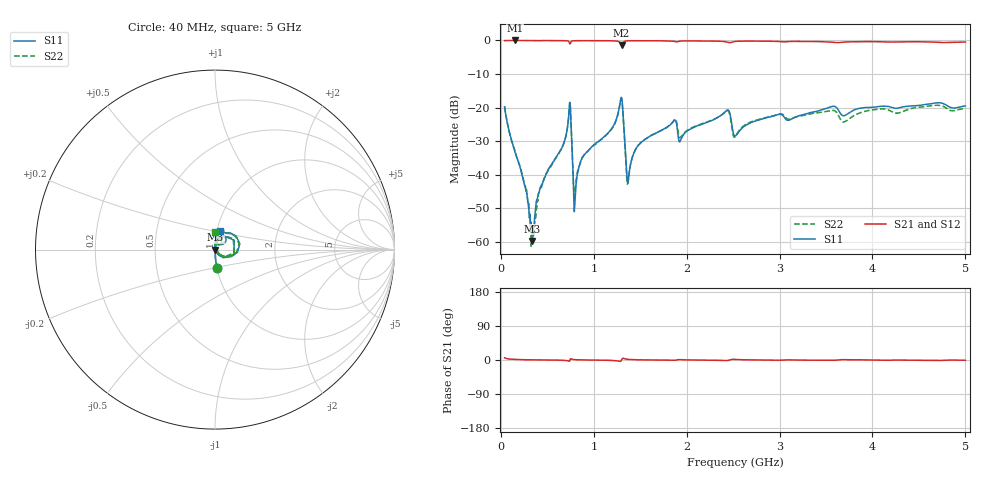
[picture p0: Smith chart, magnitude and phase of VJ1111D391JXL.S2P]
! VJ1111D391JXL
! DATE 02/15/2022  13:42
! CAPACITORS MOUNTED IN SERIES ON 25 MIL THICK MICROSTRIP SUBSTRATE
# GHz  S  MA  R  50.00
!  FREQ  S11M  S11A  S21M  S21A  S12M  S12A  S22M  S22A
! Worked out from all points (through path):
!   801 points, 40 MHz to 5 GHz, reference 50 ohm
!   highest |S21| = 0.01 dB at 151.6 MHz (marker M1); lowest = -1.3 dB at 1.299 GHz (marker M2)
!   lowest |S11| = -59.7 dB at 337.6 MHz (marker M3), VSWR 1.00, Z = 50.1 - j0.0202 ohm
!   |S11| at or under -10 dB: start of sweep to end of sweep
!   |S22| runs from -61.3 to -17.2 dB; largest |S21 - S12| = 0.01
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0.04  0.1031 -82.9  0.9949 5.8  0.9942 5.9  0.1042 -83.7
0.1516  0.02146 -86.9  1.001 1.6  0.9966 1.6  0.0229 -88.6
0.2632  0.006509 -79.8  0.9987 0.5  0.9986 0.7  0.006811 -80.6
0.3376  0.001037 -11.2  0.9964 0.4  1.001 0.4  0.00113 31.7
0.4306  0.006617 82.3  0.9957 0.2  1.001 0.1  0.006719 82.2
0.6662  0.02672 81.6  0.9948 -0.7  0.9973 -0.9  0.02681 84.9
0.7282  0.07106 64.6  0.9705 -2.8  0.9732 -2.9  0.07041 68.9
0.753  0.0665 -43.3  0.9478 3.7  0.9517 3.6  0.06664 -36.9
0.7964  0.003746 50.6  0.9924 0.9  0.9972 0.9  0.00501 42.0
0.8708  0.01736 84.2  0.9938 0.3  0.9991 0.2  0.01704 83.8
1.2986  0.1424 13.5  0.8587 -0.1  0.8635 -0.2  0.138 14.1
1.3482  0.01449 -33.7  0.9828 2.3  0.9886 2.3  0.01326 -32.9
1.373  0.008593 46.7  0.9886 1.6  0.9941 1.5  0.008468 51.7
1.466  0.02585 84.9  0.9909 0.6  0.9972 0.5  0.02597 86.7
1.6954  0.0435 84.5  0.9888 -0.1  0.9942 -0.2  0.04346 87.3
1.8628  0.0636 70.4  0.9727 -0.9  0.9776 -1.0  0.0645 75.8
1.9372  0.03314 76.2  0.9814 0.8  0.9865 0.7  0.03652 74.4
2.4332  0.09168 63.5  0.9476 -1.4  0.9522 -1.5  0.08968 65.6
2.52  0.03782 58.7  0.9676 1.5  0.9744 1.4  0.03656 68.6
3.3508  0.08522 82.2  0.966 -0.5  0.9715 -0.7  0.08162 88.7
4.1754  0.1038 70.8  0.9493 -0.6  0.957 -0.8  0.09175 84.5
5  0.106 73.7  0.9485 -0.8  0.9534 -0.9  0.09793 89.5
